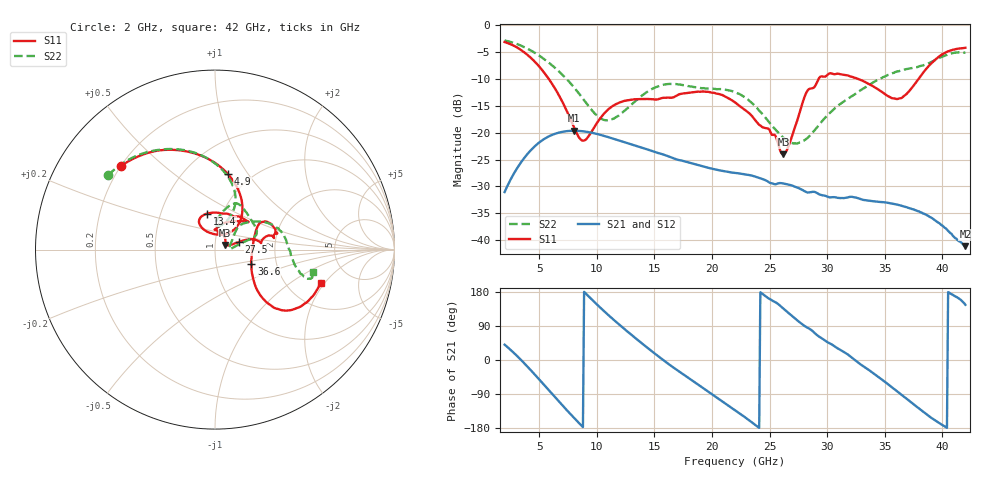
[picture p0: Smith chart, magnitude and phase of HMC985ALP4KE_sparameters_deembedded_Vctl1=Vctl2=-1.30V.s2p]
!s2p File: Measurements: S11, S21, S12, S22
# GHz S dB R 50.0
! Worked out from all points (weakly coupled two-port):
!   401 points, 2 GHz to 42 GHz, reference 50 ohm
!   highest |S21| = -19.62 dB at 8 GHz (marker M1); lowest = -41.1 dB at 42 GHz (marker M2)
!   lowest |S11| = -24.0 dB at 26.2 GHz (marker M3), VSWR 1.13, Z = 56 + j2.89 ohm
!   |S11| at or under -10 dB: 5.845 GHz to 29.25 GHz (23.4 GHz wide, 133 % of centre); 32.72 GHz to 37.92 GHz (5.206 GHz wide, 14.7 % of centre)
!   |S22| runs from -22.0 to -2.8 dB; largest |S21 - S12| = 0.00016
!   S11 on the Smith chart (normalised r, x): 2 GHz: 0.20, +0.36; 4.9 GHz: 0.79, +0.81; 13.4 GHz: 0.85, +0.35; 27.5 GHz: 1.30, +0.11; 36.6 GHz: 1.48, -0.25; 42 GHz: 3.05, -1.84
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2  -3.08 138.6  -31.06 40.5  -31.06 40.5  -2.79 145.1
3.4  -4.54 110.9  -25.59 0.9  -25.60 1.0  -3.74 122.1
4.9  -7.39 80.3  -21.99 -47.8  -22.00 -47.8  -5.46 98.6
6.2  -11.15 56.5  -20.33 -92.2  -20.34 -92.2  -7.57 80.7
8  -18.87 52.5  -19.62 -151.8  -19.63 -151.8  -11.47 65.6
8.7  -21.41 77.3  -19.70 -173.9  -19.71 -173.9  -13.37 64.9
10.8  -16.04 121.5  -20.68 124.3  -20.69 124.3  -17.67 82.9
13.4  -13.75 102.7  -22.43 56.6  -22.43 56.5  -13.99 81.2
15.4  -13.69 76.1  -23.82 8.7  -23.82 8.7  -11.27 68.6
18.9  -12.35 40.5  -26.10 -67.0  -26.11 -67.0  -11.61 42.1
22  -14.33 55.5  -27.48 -132.1  -27.50 -132.1  -12.43 19.0
24.5  -19.05 90.5  -28.72 171.8  -28.72 171.8  -16.80 12.9
26.2  -24.00 24.0  -29.46 135.6  -29.46 135.6  -20.92 3.7
27.5  -17.02 17.6  -30.29 102.2  -30.31 102.2  -21.91 7.1
28.2  -12.49 12.8  -31.07 86.8  -31.08 86.8  -21.13 16.8
28.7  -11.71 8.2  -31.02 77.2  -31.05 77.1  -20.06 24.1
31.1  -9.07 19.8  -32.17 27.4  -32.17 27.4  -14.68 44.2
33.3  -10.54 30.6  -32.59 -19.8  -32.57 -19.6  -11.56 36.1
35.4  -13.29 9.9  -33.10 -66.7  -33.12 -66.7  -9.13 23.0
36.6  -13.26 -21.4  -33.70 -95.2  -33.70 -95.2  -8.29 14.0
39.6  -5.99 -42.3  -36.69 -163.9  -36.67 -163.7  -6.23 -15.0
42  -4.16 -17.5  -41.14 145.6  -41.17 145.7  -5.06 -12.9
